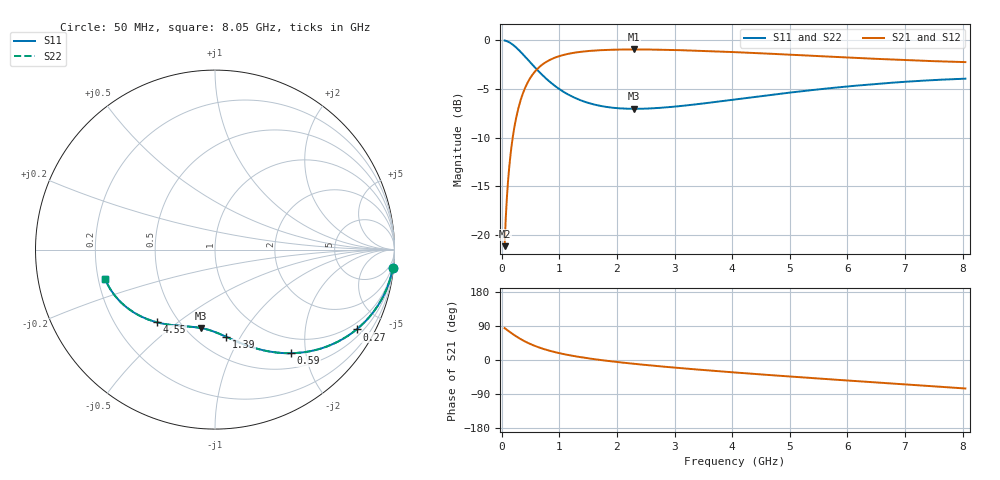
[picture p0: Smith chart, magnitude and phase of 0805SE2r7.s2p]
! AVX Thin Film Operation		Date: August 2001
! Description: Accu-P® Series, Thin Film, SMD, RF Capacitor
! Part Number: 08051J2R7ABT
! 50 MHz  -  8.05 GHz
! Serial Measurements
# mhz S db R 50
!	S11		S21		S12		S22
!	dB	Phase	dB	Phase	dB	Phase	dB	Phase
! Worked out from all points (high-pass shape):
!   401 points, 50 MHz to 8.05 GHz, reference 50 ohm
!   highest |S21| = -0.96 dB at 2.29 GHz (marker M1); lowest = -21.2 dB at 50 MHz (marker M2)
!   |S21| within 3 dB of the highest: 487.8 MHz to end of sweep
!   lowest |S11| = -7.1 dB at 2.29 GHz (marker M3), VSWR 2.60, Z = 29.8 - j32.4 ohm
!   |S11| at or under -10 dB: nowhere
!   |S22| runs from -7.1 to 0.0 dB; largest |S21 - S12| = 0
!   S11 on the Smith chart (normalised r, x): 50 MHz: 1, -20; 270 MHz: 0.74, -3.67; 590 MHz: 0.73, -1.74; 1.39 GHz: 0.68, -0.87; 4.55 GHz: 0.38, -0.42; 8.05 GHz: 0.23, -0.12
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50  -0.03 -5.8  -21.16 84.2  -21.16 84.2  -0.03 -5.8
70  -0.07 -8.1  -18.27 81.9  -18.27 81.9  -0.07 -8.1
110  -0.16 -12.7  -14.45 77.3  -14.45 77.3  -0.16 -12.7
150  -0.29 -17.1  -11.91 72.9  -11.91 72.9  -0.29 -17.1
210  -0.55 -23.5  -9.28 66.5  -9.28 66.5  -0.55 -23.5
270  -0.86 -29.4  -7.46 60.6  -7.46 60.6  -0.86 -29.4
330  -1.22 -34.9  -6.13 55.1  -6.13 55.1  -1.22 -34.9
410  -1.73 -41.5  -4.85 48.5  -4.85 48.5  -1.73 -41.5
590  -2.89 -53.6  -3.13 36.3  -3.13 36.3  -2.89 -53.7
750  -3.83 -62.0  -2.32 28.0  -2.32 28.0  -3.83 -62.0
930  -4.73 -69.4  -1.79 20.6  -1.79 20.6  -4.73 -69.4
1130  -5.51 -76.0  -1.44 14.0  -1.44 14.0  -5.51 -76.0
1390  -6.22 -82.9  -1.19 7.0  -1.19 7.0  -6.22 -82.9
1790  -6.83 -91.4  -1.01 -1.4  -1.01 -1.4  -6.83 -91.4
2290  -7.05 -99.9  -0.96 -10.0  -0.96 -10.0  -7.05 -99.9
2730  -6.96 -106.3  -0.98 -16.4  -0.98 -16.4  -6.96 -106.4
3370  -6.59 -114.7  -1.08 -24.8  -1.08 -24.8  -6.59 -114.8
4050  -6.09 -122.8  -1.23 -32.9  -1.23 -32.9  -6.09 -122.9
4550  -5.72 -128.5  -1.36 -38.6  -1.36 -38.6  -5.72 -128.5
5390  -5.13 -137.6  -1.60 -47.7  -1.60 -47.7  -5.13 -137.6
6730  -4.39 -151.5  -1.98 -61.6  -1.98 -61.6  -4.39 -151.5
8050  -3.96 -165.0  -2.26 -75.2  -2.26 -75.2  -3.96 -165.0
